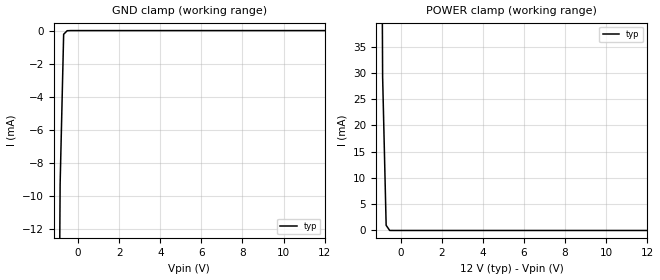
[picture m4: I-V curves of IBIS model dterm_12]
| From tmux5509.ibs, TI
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| dterm_12
[Model]   dterm_12
Model_type   Terminator
|   typ   min   max
C_comp   4.014581e-12   NA   NA
[Voltage Range]   12   NA   NA
[Temperature Range]   27   NA   NA
[Power Clamp Reference]   12   NA   NA
[GND Clamp Reference]   0   NA   NA
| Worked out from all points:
|   GND clamp passes 1 mA (typ) near -0.72 V on its own axis
|   POWER clamp passes 1 mA (typ) near -0.71 V on its own axis
[GND Clamp]
|   Voltage   I(typ)   I(min)   I(max)
-5V       -2.839A    NA         NA
-1.051V   -42.72mA   NA         NA
-878.8mV  -9.288mA   NA         NA
-707.1mV  -223.6uA   NA         NA
-535.4mV  -9.048uA   NA         NA
12V       1.089nA    NA         NA
[POWER Clamp]
|   Voltage   I(typ)   I(min)   I(max)
-5V       7.431A     NA         NA
-1.05V    166.5mA    NA         NA
-878.8mV  29.29mA    NA         NA
-707.1mV  982.9uA    NA         NA
-535.4mV  4.821uA    NA         NA
12V       -934pA     NA         NA
